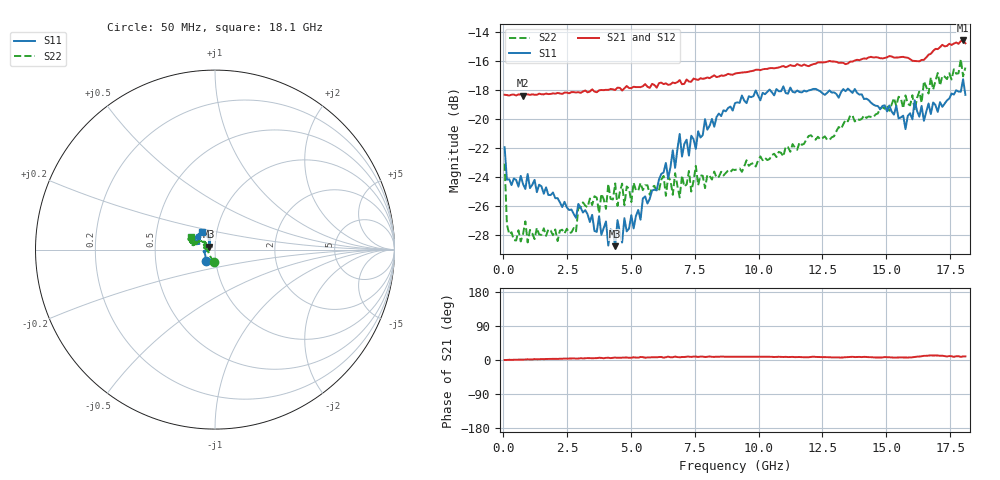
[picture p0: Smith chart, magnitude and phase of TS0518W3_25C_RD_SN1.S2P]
! Network Analyzer HP8720D.06.14 Serial No. US36140669
! 17 Jun 2005  09:13:37
! Frequency  S11  S21  S12  S22
# HZ  S  DB R 50
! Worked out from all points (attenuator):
!   201 points, 50 MHz to 18.1 GHz, reference 50 ohm
!   highest |S21| = -14.58 dB at 18.01 GHz (marker M1); lowest = -18.4 dB at 772 MHz (marker M2)
!   lowest |S11| = -28.8 dB at 4.382 GHz (marker M3), VSWR 1.08, Z = 46.8 + j1.46 ohm
!   |S11| at or under -10 dB: start of sweep to end of sweep
!   |S22| runs from -28.5 to -15.9 dB; largest |S21 - S12| = 0.0053
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5e7  -21.96 -130.0  -18.34 -0.1  -18.33 -0.1  -23.09 -95.6
1.4025e8  -24.20 -152.3  -18.36 0.1  -18.37 0.2  -27.30 -136.8
2.305e8  -24.18 -158.3  -18.39 0.6  -18.37 0.4  -27.98 -151.7
7.72e8  -24.51 -166.1  -18.40 1.2  -18.34 1.1  -27.96 -177.0
2.12575e9  -25.48 -173.8  -18.21 2.9  -18.25 3.0  -28.45 169.3
3.1185e9  -26.48 -179.4  -18.11 4.3  -18.14 4.3  -25.78 173.5
4.382e9  -28.80 154.6  -18.01 6.4  -17.92 5.8  -24.46 169.8
4.47225e9  -27.00 148.4  -17.84 5.9  -17.92 6.4  -26.02 172.8
4.65275e9  -28.55 143.0  -18.04 6.1  -17.89 6.3  -24.48 172.7
4.743e9  -26.86 146.0  -17.89 6.4  -17.93 6.5  -25.97 168.2
6.09675e9  -24.19 120.2  -17.54 7.8  -17.52 7.7  -24.97 162.6
6.7285e9  -23.39 120.5  -17.54 9.1  -17.61 8.3  -23.75 156.7
6.909e9  -21.04 117.3  -17.32 7.1  -17.48 7.4  -25.43 151.9
7.27e9  -22.54 114.1  -17.43 9.0  -17.41 8.0  -23.60 153.9
9.075e9  -18.91 126.6  -16.88 8.8  -16.88 8.8  -23.54 145.9
1.21435e10  -17.93 154.2  -16.22 8.8  -16.21 8.6  -21.32 146.5
1.512175e10  -19.08 158.7  -15.66 7.1  -15.65 7.6  -19.45 160.2
1.57535e10  -20.71 159.6  -15.76 6.6  -15.81 6.3  -18.38 157.9
1.61145e10  -18.72 155.0  -16.00 8.0  -16.02 7.6  -19.43 163.8
1.64755e10  -20.14 152.9  -15.92 10.9  -15.84 11.4  -17.41 161.5
1.800975e10  -17.26 125.8  -14.58 9.4  -14.76 9.5  -17.06 160.1
1.81e10  -18.35 127.7  -14.78 9.5  -14.81 8.0  -16.46 153.3
